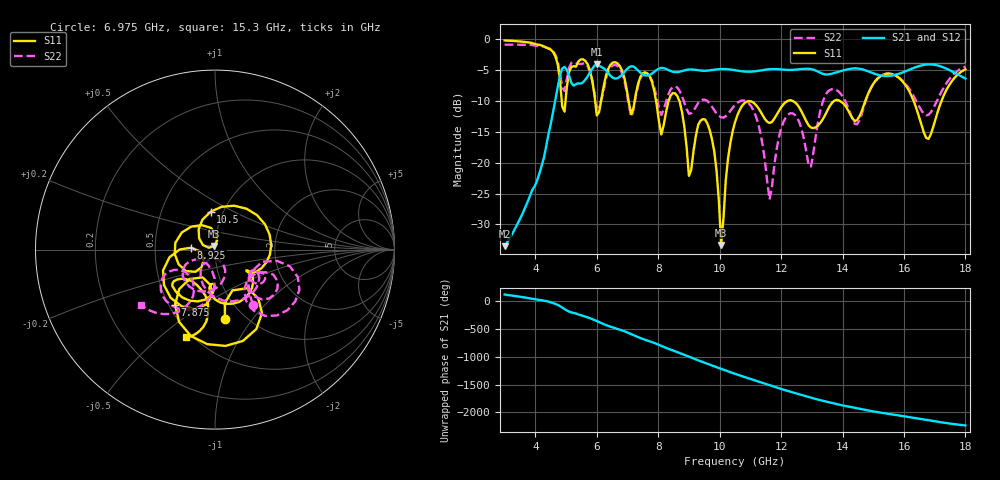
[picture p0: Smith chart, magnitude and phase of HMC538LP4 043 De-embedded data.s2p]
! Chelmsford, MA 01824
! http://www.hittite.com
! Tel: 978-250-3343
! Fax: 978-250-3373
! Device  :  HMC538LP4
! Description:  600 Analog Phase Shifter
! Frequency  :  6.0 GHz - 15.0 GHz
! Package  :  LP4  - 4x4 mm Quad Flatpack No-Lead (QFN) Plastic Package: 24 pin
! Ports  :  2 RF, 1 DC
!  Pin  3  = Rfin  = Port 1
!  Pin  16  = Rfout = Port 2
!  pin  21  = vCTL
! Voltages:  VCTL  = 0 to 5.0 Volts
! Currents :  Vb(V)  Vd(V)  Ib(mA)  Id(mA)
!  0.00  4.30  0.000000	0.474918
! Data:  The device was measured on evaluation board 111296-1.
!  Data was collected using a calibrated network analyzer.
!  The evaluation circuit board was modeled and simulated.This was use
!  to removed the evaluation board circuit from the measured data.
!  The reference plane is the center of the package pin.
! Misc:  Lot #
!Date Measured:  03 - 11 -2009
! Date:  03 - 17 -2009
! Note:
!  Hittite Microwave supplies this data as a sample of measured data at the
!  package pin for this package product.  Your particular data for this product
!  may vary.
!  Data was taken at 25 degrees C.
!  Hittite Microwave reserves the right to change this data at anytime.
# MHz S MA R 50
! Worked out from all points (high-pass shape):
!   201 points, 3 GHz to 18 GHz, reference 50 ohm
!   highest |S21| = -4.07 dB at 6 GHz (marker M1); lowest = -33.5 dB at 3 GHz (marker M2)
!   |S21| within 3 dB of the highest: 4.756 GHz to 5.173 GHz (417 MHz wide, 8.4 % of centre); 5.521 GHz to end of sweep
!   lowest |S11| = -33.3 dB at 10.05 GHz (marker M3), VSWR 1.04, Z = 49.4 + j2.06 ohm
!   |S11| at or under -10 dB: 8.69 GHz to 12.21 GHz (3.523 GHz wide, 33.7 % of centre); 12.38 GHz to 13.72 GHz (1.338 GHz wide, 10.3 % of centre); 16.31 GHz to 17.22 GHz (908.5 MHz wide, 5.42 % of centre)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
!   |S22| runs from -26.0 to -0.9 dB; largest |S21 - S12| = 0.0025
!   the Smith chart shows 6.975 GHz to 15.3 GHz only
!   S11 on the Smith chart (normalised r, x): 6.975 GHz: 0.81, -0.74; 7.875 GHz: 0.54, -0.39; 8.925 GHz: 0.76, +0.02; 10.5 GHz: 0.87, +0.39; 15.3 GHz: 0.47, -0.62
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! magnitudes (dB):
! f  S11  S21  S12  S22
! 3 GHz  -0.2  -33.5  -33.5  -0.9
! 4.575 GHz  -2.0  -11.9  -11.9  -1.9
! 4.875 GHz  -10.9  -4.7  -4.8  -7.8
! 5.55 GHz  -3.2  -7.0  -7.0  -3.9
! 6 GHz  -12.3  -4.1  -4.1  -11.0
! 6.975 GHz  -8.1  -4.9  -4.9  -8.6
! 7.875 GHz  -8.4  -5.3  -5.3  -7.9
! 8.025 GHz  -13.3  -4.8  -4.8  -11.2
! 8.55 GHz  -8.8  -5.3  -5.3  -7.6
! 8.925 GHz  -17.5  -4.9  -5.0  -11.3
! 9.6 GHz  -13.6  -5.1  -5.1  -10.0
! 10.05 GHz  -33.3  -4.8  -4.8  -12.6
! 10.5 GHz  -13.4  -5.0  -5.0  -10.6
! 11.18 GHz  -10.6  -5.2  -5.2  -12.4
! 11.62 GHz  -13.6  -4.8  -4.9  -26.0
! 12.22 GHz  -10.0  -5.0  -5.0  -12.2
! 13.05 GHz  -14.4  -4.9  -4.9  -18.4
! 13.5 GHz  -11.6  -5.7  -5.7  -8.6
! 15.3 GHz  -5.8  -5.9  -5.9  -5.8
! 15.53 GHz  -5.6  -5.9  -5.9  -5.6
! 16.8 GHz  -16.1  -4.1  -4.1  -12.2
! 18 GHz  -4.9  -6.4  -6.4  -4.4
